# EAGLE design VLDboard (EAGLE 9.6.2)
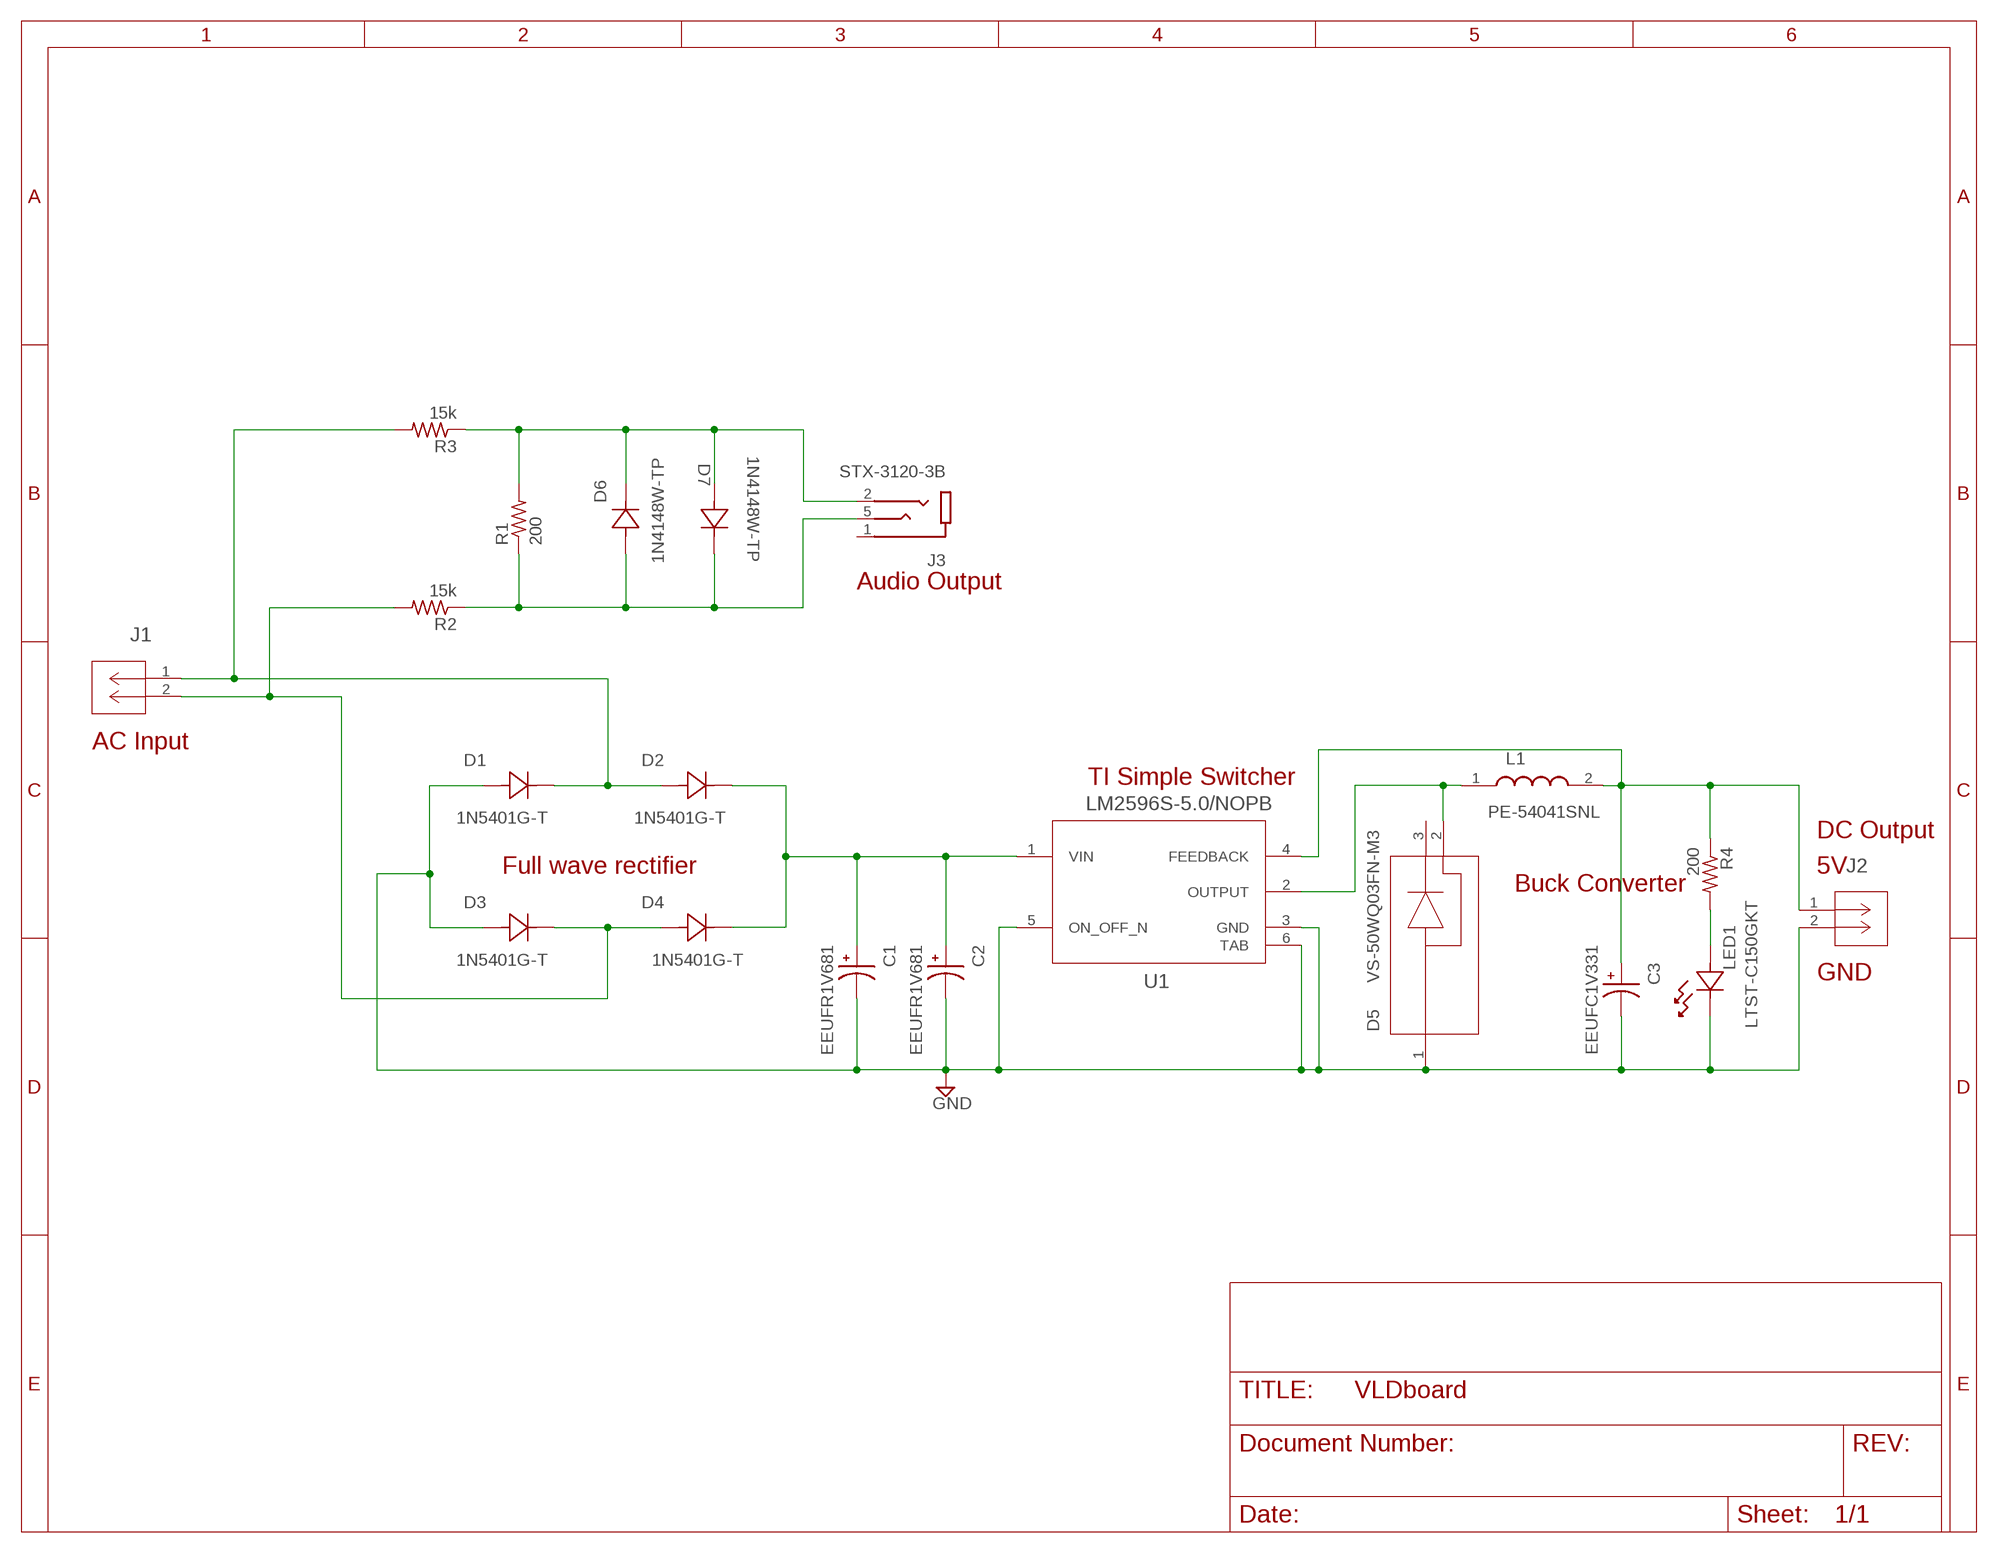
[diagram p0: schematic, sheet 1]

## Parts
C1  EEUFR1V681  [CAPPRD500W60D1000H2000]
C2  EEUFR1V681  [CAPPRD500W60D1000H2000]
C3  EEUFC1V331  [CAPPRD500W60D1000H1600]
D1  1N5401G-T  [DO-201AD_DIO]
D2  1N5401G-T  [DO-201AD_DIO]
D3  1N5401G-T  [DO-201AD_DIO]
D4  1N5401G-T  [DO-201AD_DIO]
D5  VS-50WQ03FN-M3  [D-PAK_TO252AA_M_VIS]
D6  1N4148W-TP  [SOD123_MCC]
D7  1N4148W-TP  [SOD123_MCC]
J1  1935161  [CONN_1935161_PXC]
J2  1935161  [CONN_1935161_PXC]
J3  STX-3120-3B  [KYCON_STX-3120-3B]
L1  PE-54041SNL  [P0846SNLT]
LED1  LTST-C150GKT  [LED_LTST-C150GKT_LTO]
R1  200  R-US_R1206  [R1206]
R2  15k  R-US_R1206  [R1206]
R3  15k  R-US_R1206  [R1206]
R4  200  R-US_R1206  [R1206]
U1  LM2596S-5.0/NOPB  [KTT0005B]

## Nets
GND: C1.N C2.N C3.N D1.2 D3.2 D5.1 J2.2 LED1.1 U1.3(GND) U1.5(ON_OFF_N) U1.6(TAB)
N$1: D1.1 D2.2 J1.1 R3.2
N$2: D5.2 L1.1 U1.2(OUTPUT)
N$3: C3.P J2.1 L1.2 R4.1 U1.4(FEEDBACK)
N$4: C1.P C2.P D2.1 D4.1 U1.1(VIN)
N$5: D3.1 D4.2 J1.2 R2.2
N$6: D6.1 D7.2 J3.2 R1.2 R3.1
N$7: D6.2 D7.1 J3.5 R1.1 R2.1
N$9: LED1.2 R4.2
Unconnected: D5.3 J3.1

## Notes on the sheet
- Audio Output
- AC Input
- TI Simple Switcher
- DC Output
- Full wave rectifier
- 5V
- Buck Converter
- GND

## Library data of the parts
C1 C2 = VLD5V_ExtractionCircuit:EEUFR1V681: FR-A Check availability; AVAILABILITY: In Stock; DESCRIPTION: Cap Aluminum Lytic 680uF 35V 20% (10 X 20mm) Radial 5mm 2180mA 10000h 105°C Bulk; MF: Panasonic; MP: EEUFR1V681; PACKAGE: RADIAL-2 Panasonic; PRICE: None; PURCHASE-URL: https://pricing.snapeda.com/search/part/EEUFR1V681/?ref=eda
C3 = VLD5V_ExtractionCircuit:EEUFC1V331: FC-A Check availability; AVAILABILITY: In Stock; DESCRIPTION: Cap Aluminum 330uF 35V 20% (10 X 16mm) Radial 5mm 1050mA 3000 hr 105C Bulk; MF: Panasonic Electronic; MP: EEU-FC1V331; PACKAGE: RADIAL-2 Panasonic; PRICE: None; PURCHASE-URL: https://pricing.snapeda.com/search/part/EEU-FC1V331/?ref=eda
D1-D4 = VLD5V_ExtractionCircuit:1N5401G-T; COPYRIGHT: Copyright (C) 2022 Ultra Librarian. All rights reserved.; MANUFACTURER_PART_NUMBER: 1N5401G-T; MFR_NAME: Diodes Inc
D5 = VLD5V_ExtractionCircuit:VS-50WQ03FN-M3; COPYRIGHT: Copyright (C) 2022 Ultra Librarian. All rights reserved.; MANUFACTURER_PART_NUMBER: VS-50WQ03FN-M3; MFR_NAME: Vishay
D6 D7 = VLD5V_ExtractionCircuit:1N4148W-TP; COPYRIGHT: Copyright (C) 2022 Ultra Librarian. All rights reserved.; MANUFACTURER_PART_NUMBER: 1N4148W-TP; MFR_NAME: MCC
J1 J2 = VLD5V_ExtractionCircuit:1935161; COPYRIGHT: Copyright (C) 2022 Ultra Librarian. All rights reserved.; MANUFACTURER_PART_NUMBER: 1935161; MFR_NAME: Phoenix Contact
J3 = VLD5V_ExtractionCircuit:STX-3120-3B: Check availability; AVAILABILITY: In Stock; DESCRIPTION: 3.50mm (0.141, 1/8, Mini Plug) - Headphone Phone Jack Stereo (3 Conductor, TRS) Connector Kinked Pin; MF: Kycon; MP: STX-3120-3B; PACKAGE: None; PRICE: None; PURCHASE-URL: https://pricing.snapeda.com/search/part/STX-3120-3B/?ref=eda
L1 = VLD5V_ExtractionCircuit:PE-54041SNL: Fixed Inductors SIMPLE SWITCHER IND; ARROW_PART_NUMBER: PE-54041SNL; ARROW_PRICE-STOCK: https://www.arrow.com/en/products/pe-54041snl/pulse-electronics-corporation?region=nac; DESCRIPTION: Fixed Inductors SIMPLE SWITCHER IND; HEIGHT: 9mm; MANUFACTURER_NAME: Pulse; MANUFACTURER_PART_NUMBER: PE-54041SNL; MOUSER_PART_NUMBER: 673-PE-54041SNL; MOUSER_PRICE-STOCK: https://www.mouser.co.uk/ProductDetail/Pulse-Electronics/PE-54041SNL?qs=HTH0j2vZhnATbaPjpCjZKw%3D%3D
LED1 = VLD5V_ExtractionCircuit:LTST-C150GKT; COPYRIGHT: Copyright (C) 2022 Ultra Librarian. All rights reserved.; MANUFACTURER_PART_NUMBER: LTST-C150GKT; MFR_NAME: LITE-ON
R1-R4 = rcl:R-US_: RESISTOR, American symbol; SPICEPREFIX: R
U1 = VLD5V_ExtractionCircuit:LM2596S-5.0/NOPB; COPYRIGHT: Copyright (C) 2022 Ultra Librarian. All rights reserved.; MANUFACTURER_PART_NUMBER: LM2596S-5.0/NOPB; MFR_NAME: Texas Instruments; REFDES: RefDes; TYPE: TYPE

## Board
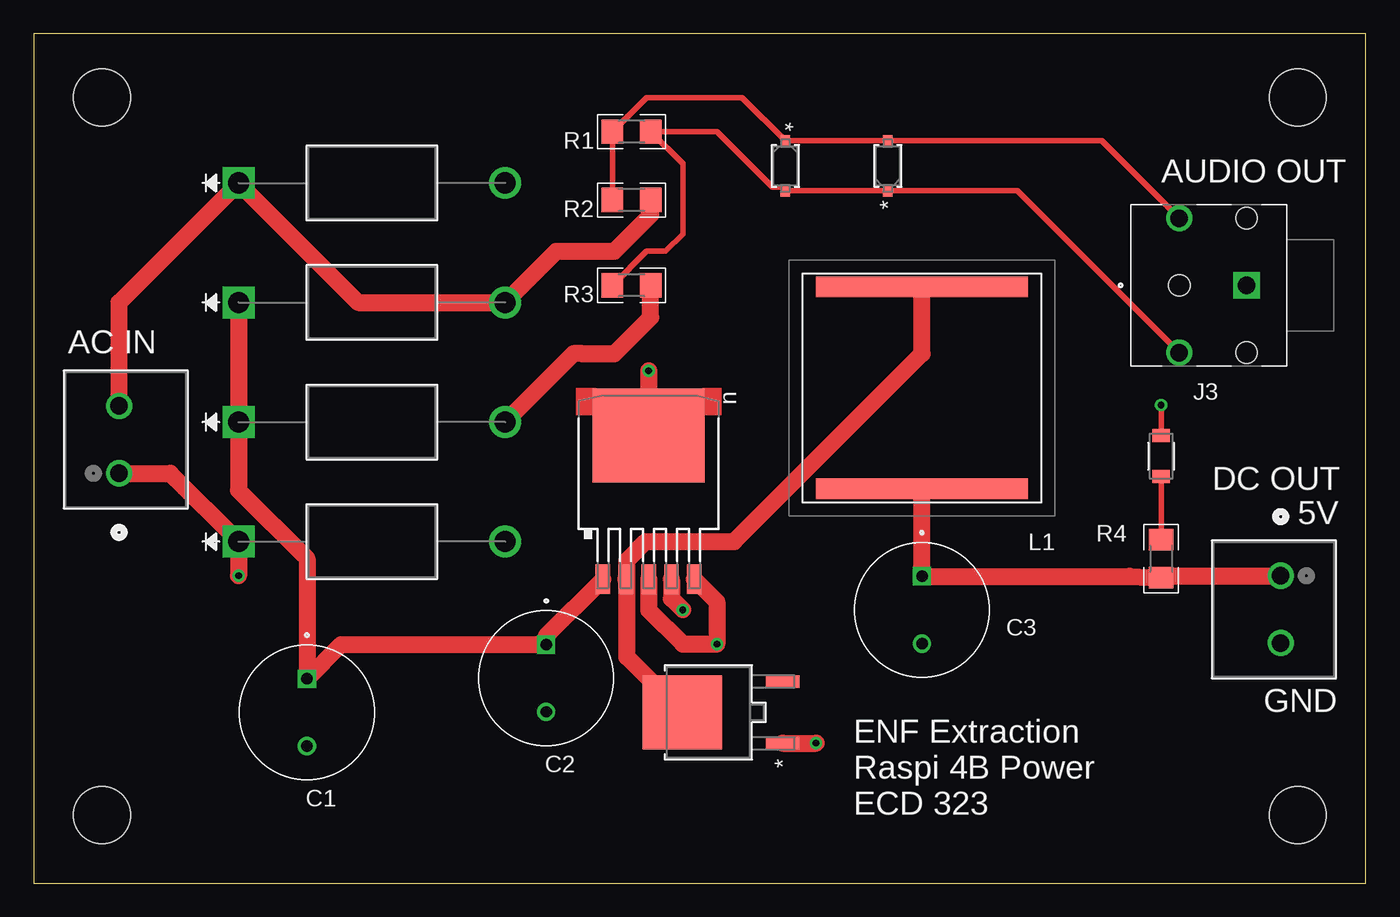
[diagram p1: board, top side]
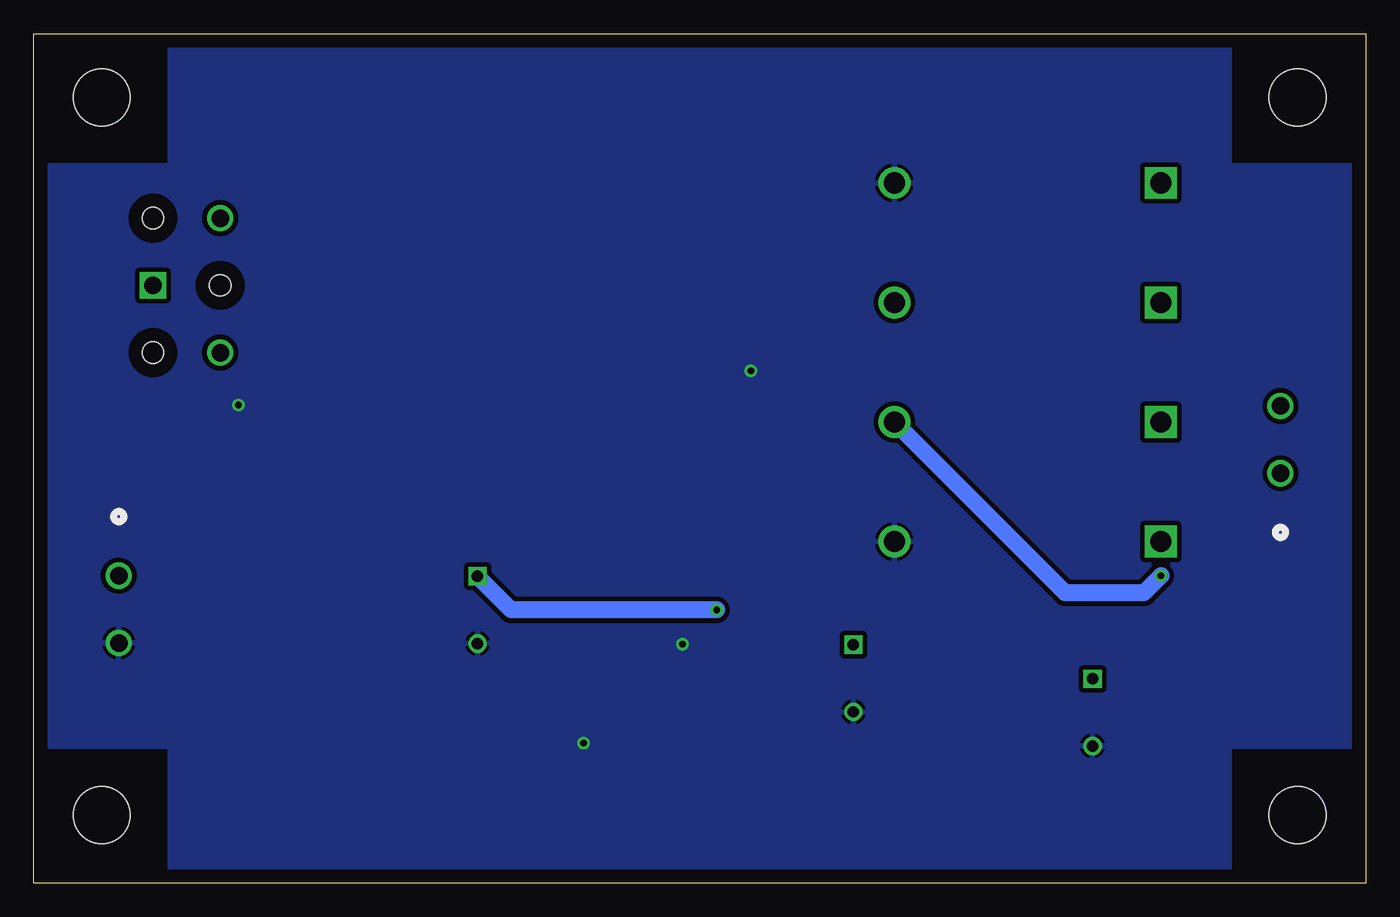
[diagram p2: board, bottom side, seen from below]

Size 99.04 x 63.17 mm. Coordinates in mm from the lower left corner, seen from the top.
Outline: 0,0 99.04,0 99.04,63.17 0,63.17 0,0
Copper layers (1*16): Top 0.035mm / dielectric 1.5mm / Bottom 0.035mm
Design rules "default *": minimum track width 6mil, minimum drill 0.35mm, track to track 14mil, track to pad 14mil, pad to pad 14mil, via to via 14mil, smd to smd 14mil, copper to edge 40mil, drill to drill 20mil, minimum pad ring 10mil, minimum via ring 8mil, stop-mask expansion 4mil, vias tented up to drill 0mil, thermal gap 10mil
Holes 4.24 mm at 5.08,58.42 5.08,5.08 93.98,5.08 93.98,58.42

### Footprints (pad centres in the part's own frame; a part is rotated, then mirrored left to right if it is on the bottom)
CAPPRD500W60D1000H2000 = drill 0.85 pad 1.2: N 2.5,0 | drill 0.85 pad 1.2 square: P -2.5,0
CAPPRD500W60D1000H1600 = drill 0.85 pad 1.2: N 2.5,0 | drill 0.85 pad 1.2 square: P -2.5,0
DO-201AD_DIO = drill 1.575 pad 2.083 square: 1 0,0 | drill 1.575 pad 2.083: 2 19.812,0
D-PAK_TO252AA_M_VIS = smd 0.94 x 2.489: 1 -2.29,-5.524; 3 2.29,-5.524 | smd 5.512 x 5.918: 2 0,1.956
SOD123_MCC = smd 0.864 x 0.711: 1 -1.854,0; 2 1.854,0
CONN_1935161_PXC = drill 1.295 pad 1.803: 1 0,0; 2 5.004,0
KYCON_STX-3120-3B = drill 1.3 square: 1 0,0 | drill 1.3: 2 5,5; 5 5,-5 | hole 1.6: 0,5; 0,-5; 5,0
P0846SNLT = smd 1.52 x 15.75: 1 -7.495,0; 2 7.495,0
LED_LTST-C150GKT_LTO = smd 0.965 x 1.295: 1 -1.524,0; 2 1.524,0
R1206 = smd 1.6 x 1.803: 1 -1.422,0; 2 1.422,0
KTT0005B = smd 2.16 x 1.07: 1 5.338,-3.4; 2 5.338,-1.7; 3 5.338,0.005; 4 5.338,1.7; 5 5.338,3.4 | smd 6.99 x 8.33: 6 -5.338,0

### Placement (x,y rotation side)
C1  20.32,12.7 270 top
C2  38.1,15.24 270 top
C3  66.04,20.32 270 top
D1  15.24,25.4 0 top
D2  15.24,34.29 0 top
D3  15.24,52.07 0 top
D4  15.24,43.18 0 top
D5  50.16,12.7 90 top
D6  63.5,53.34 90 top
D7  55.88,53.34 270 top
J1  6.35,30.48 90 top
J2  92.71,22.86 270 top
J3  90.17,44.45 180 top
L1  66.04,36.83 270 top
LED1  83.82,31.75 270 top
R1  44.45,55.88 0 top
R2  44.45,50.8 0 top
R3  44.45,44.45 0 top
R4  83.82,24.13 90 top
U1  45.72,27.94 270 top

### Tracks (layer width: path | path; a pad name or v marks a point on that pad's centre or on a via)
GND  (via drill 0.51)
  Top 0.406: LED1.1 v83.82,35.56
  Top 1.27: U1.3 45.73,20.32 48.26,17.78 v50.8,17.78 50.8,20.92 U1.5 | v45.72,38.1 45.72,35.56 46.86,34.42 U1.6 | D5.1 v58.17,10.41
  pour Bottom: -3.81,53.34 10.16,53.34 10.16,67.31 87.63,67.31 88.9,67.31 88.9,53.34 102.87,53.34 102.87,10.16 88.9,10.16 88.9,-3.81 10.16,-3.81 10.16,10.16 -3.81,10.16
N$1  (via drill 0.51)
  Top 1.27: J1.1 10.16,30.48 D1.1 v15.24,22.86 | D2.2 40.13,39.37 40.79,39.37 43.18,39.37 45.87,42.06 R3.2
  Bottom 1.27: v15.24,22.86 16.51,21.59 22.35,21.59 D2.2
N$2
  Top 1.27: L1.1 66.04,39.37 52.07,25.4 45.51,25.4 44.1,23.99 44.1,22.68 | U1.2 44.1,22.68 | D5.2 44.1,16.81 44.1,22.68
N$3  (via drill 0.51)
  Top 1.27: L1.2 C3.P 81.47,22.82 R4.1 83.97,22.86 J2.1 | U1.4 47.42,21.16 v48.26,20.32
  Bottom 1.27: C3.P 63.54,20.32 v48.26,20.32
N$4
  Top 1.27: D4.1 D2.1 15.24,29.21 20.32,24.13 C1.P 22.86,17.74 C2.P 38.1,18.38 U1.1
N$5
  Top 1.27: J1.2 6.35,43.18 D3.1 24.13,43.18 D4.2 38.86,46.99 43.18,46.99 45.87,49.68 R2.2
N$6
  Top 0.406: R3.1 45.57,46.99 46.99,46.99 48.26,48.26 48.26,53.49 R1.2 50.81,55.88 54.94,51.75 55.61,51.75 D7.2 D6.1 73.13,51.49 J3.2
N$7
  Top 0.406: J3.5 79.43,55.19 D6.2 D7.1 52.65,58.42 45.57,58.42 R1.1 R2.1
N$9
  Top 0.406: LED1.2 R4.2

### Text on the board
tPlace: AUDIO OUT | AC IN | DC OUT | 5V | GND
tNames: ENF Extraction / Raspi 4B Power / ECD 323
